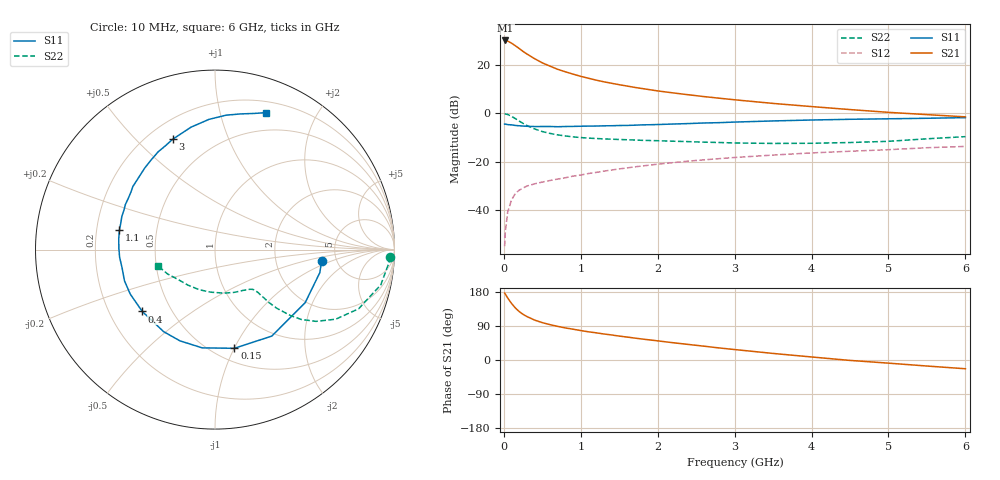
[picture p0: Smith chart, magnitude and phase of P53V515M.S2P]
! SIEMENS Small Signal Semiconductors
! BFP183
! Si NPN RF Bipolar Junction Transistor in SOT143
! VCE = 3.5 V  IC = 15 mA
! Common Emitter S-Parameters:  March  1996
# GHz  S  MA  R  50
!  f  S11  S21  S12  S22
! GHz  MAG  ANG  MAG  ANG  MAG  ANG  MAG  ANG
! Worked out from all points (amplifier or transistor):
!   36 points, 10 MHz to 6 GHz, reference 50 ohm
!   highest |S21| = 30.1 dB at 20 MHz (marker M1)
!   |S21| within 3 dB of that: start of sweep to 185.4 MHz
!   unconditionally stable (mu >= 1): 959.6 MHz to 5.568 GHz
!   at 250 MHz: K = 0.41, MSG = 28.2 dB, |S12| = -30.9 dB
!   at 1.4 GHz: K = 1.11, MAG = 15.9 dB, |S12| = -23.4 dB
!   at 6 GHz: K = 0.94, MSG = 6.1 dB, |S12| = -13.7 dB
!   S11 on the Smith chart (normalised r, x): 10 MHz: 3.82, -0.73; 150 MHz: 0.62, -1.00; 400 MHz: 0.34, -0.33; 1.1 GHz: 0.30, +0.09; 3 GHz: 0.30, +0.65; 6 GHz: 0.31, +1.39
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0.01  0.5976 -5.9  31.91 176.6  0.0018 83.8  0.9774 -2.4
0.02  0.5979 -12.4  31.93 173.6  0.0037 84.4  0.9696 -4.8
0.05  0.583 -30.4  31.05 163.6  0.0091 79.5  0.9445 -12.0
0.1  0.5764 -56.7  28.04 149.2  0.0163 67.3  0.8655 -22.4
0.15  0.5604 -78.9  24.81 137.2  0.0221 58.5  0.776 -30.0
0.2  0.5521 -97.4  21.75 127.8  0.0258 54.4  0.6901 -35.4
0.25  0.5447 -111.0  18.95 120.4  0.0286 50.7  0.6183 -39.0
0.3  0.5392 -122.1  16.77 114.7  0.0314 48.1  0.5596 -41.1
0.4  0.5319 -139.6  13.41 105.3  0.0349 46.0  0.4752 -43.5
0.5  0.5333 -152.3  11.01 98.6  0.038 45.5  0.4198 -44.5
0.6  0.5335 -161.0  9.411 93.3  0.0409 46.7  0.384 -44.6
0.7  0.5276 -168.9  8.095 88.7  0.0438 47.2  0.3581 -44.9
0.9  0.5359 179.0  6.438 81.3  0.0504 48.4  0.3262 -45.3
1.1  0.5435 168.6  5.29 74.4  0.057 49.1  0.3069 -46.4
1.5  0.559 153.2  3.893 63.1  0.071 49.4  0.2874 -50.5
1.8  0.577 142.5  3.241 55.3  0.0816 48.6  0.2763 -55.2
2.2  0.5997 130.8  2.637 45.6  0.0957 46.4  0.2649 -62.6
3  0.6584 111.0  1.9 27.6  0.1222 40.7  0.2439 -81.7
3.5  0.695 101.1  1.599 17.3  0.1371 36.8  0.2384 -95.9
4.5  0.7515 85.3  1.193 -1.1  0.1644 28.4  0.2488 -127.4
5.5  0.7887 74.1  0.939 -15.9  0.1944 20.9  0.2971 -152.8
6  0.8133 69.7  0.844 -23.1  0.2068 16.4  0.3293 -163.9
